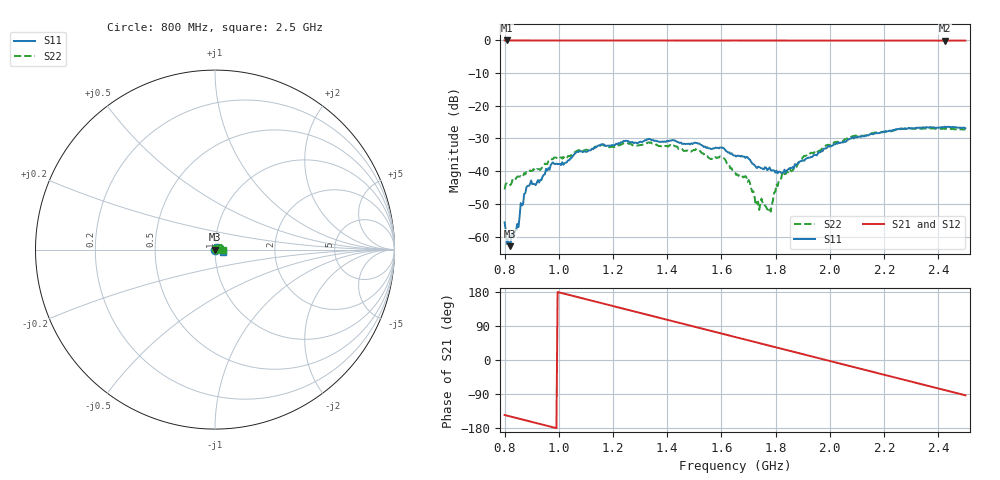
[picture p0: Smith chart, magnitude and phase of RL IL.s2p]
!Agilent Technologies,N5234A,MY52241180,A.10.00.00
!Agilent N5234A: A.10.00.00
!Date: Tuesday, August 18, 2015 23:49:29
!Correction: S11(Full 2 Port(1,2))
!S21(Full 2 Port(1,2))
!S12(Full 2 Port(1,2))
!S22(Full 2 Port(1,2))
!S2P File: Measurements: S11, S21, S12, S22:
# Hz S  dB  R 50
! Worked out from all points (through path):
!   401 points, 800 MHz to 2.5 GHz, reference 50 ohm
!   highest |S21| = -0.15 dB at 808.5 MHz (marker M1); lowest = -0.2 dB at 2.424 GHz (marker M2)
!   group delay of S21, straight-line fit = 503 ps
!   lowest |S11| = -62.8 dB at 821.2 MHz (marker M3), VSWR 1.00, Z = 49.9 - j0.0525 ohm
!   |S11| at or under -10 dB: start of sweep to end of sweep
!   |S22| runs from -52.3 to -26.9 dB; largest |S21 - S12| = 0.0031
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8e8  -55.53 -146.2  -0.15 -145.2  -0.16 -145.2  -45.49 49.9
8.085e8  -62.08 162.7  -0.15 -146.7  -0.16 -146.7  -43.69 53.8
8.2125e8  -62.79 -133.6  -0.15 -149.0  -0.16 -149.0  -44.17 50.3
8.425e8  -57.96 99.8  -0.15 -152.9  -0.16 -152.9  -42.10 47.2
8.68e8  -50.05 86.1  -0.15 -157.5  -0.17 -157.5  -41.57 51.9
8.8925e8  -44.43 96.6  -0.15 -161.4  -0.16 -161.3  -40.21 62.2
9.2325e8  -42.66 68.6  -0.16 -167.5  -0.16 -167.5  -39.35 54.8
9.785e8  -37.30 76.7  -0.16 -177.5  -0.16 -177.5  -36.22 57.6
1.08475e9  -33.97 49.7  -0.16 163.3  -0.18 163.2  -33.34 43.2
1.24625e9  -30.70 19.0  -0.16 133.9  -0.17 133.9  -31.37 25.1
1.3695e9  -30.97 -5.9  -0.17 111.6  -0.18 111.6  -32.33 3.9
1.60325e9  -32.78 -60.8  -0.17 69.2  -0.18 69.2  -35.70 -28.8
1.65e9  -35.20 -80.3  -0.17 60.8  -0.18 60.8  -40.23 -24.5
1.69675e9  -35.75 -94.6  -0.17 52.3  -0.19 52.3  -43.20 -28.8
1.735e9  -38.59 -117.5  -0.18 45.4  -0.19 45.3  -49.24 3.2
1.77325e9  -39.34 -133.2  -0.18 38.4  -0.19 38.4  -51.70 34.6
1.82e9  -40.42 173.8  -0.18 30.0  -0.19 29.9  -42.26 76.9
1.93475e9  -35.61 115.2  -0.19 9.2  -0.19 9.1  -34.35 75.1
2.075e9  -30.07 67.9  -0.20 -16.2  -0.21 -16.2  -29.82 57.7
2.2195e9  -27.64 36.8  -0.19 -42.4  -0.22 -42.4  -27.80 38.4
2.4235e9  -26.40 -6.3  -0.22 -79.4  -0.22 -79.4  -27.03 5.8
2.5e9  -26.90 -18.4  -0.21 -93.2  -0.23 -93.2  -27.27 -4.5
